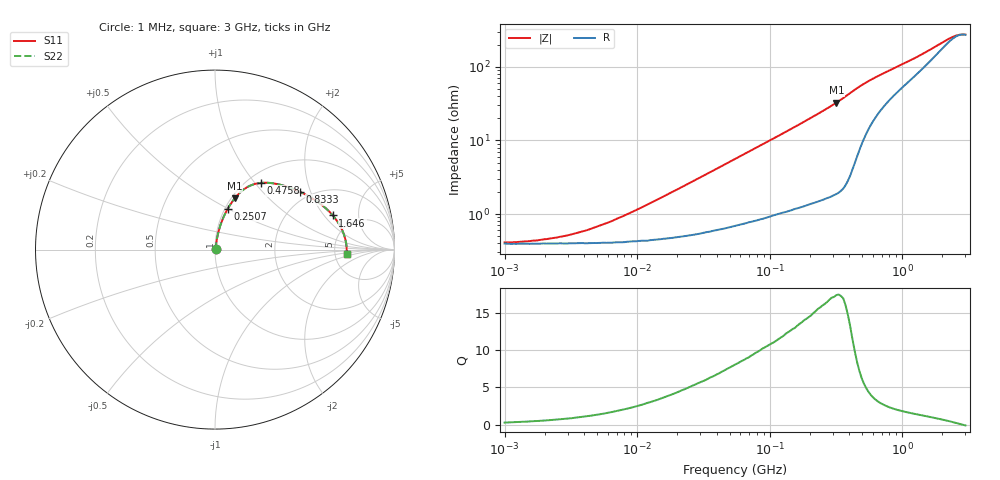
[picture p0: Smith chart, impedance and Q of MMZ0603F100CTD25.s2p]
! S-Parameter Data Generated by TDK Corporation
! Copyright(C) 2025 TDK Corporation.
! All Rights Reserved.
! TDK P/N: MMZ0603F100CTD25 (Chip Bead)
! Property: |Z|=10ohm at 100MHz
! Size(LxWxT): 0.6x0.3x0.3mm
! Model Type: s2p (Touchstone File Format Version 1.0)
! Frequency: DC=Yes Start=1MHz Stop=3000MHz 202points Log-sweep
! Model Generated on Feb. 6, 2025
! Terms and conditions regarding TDK Simulation Models:
! 1)This simulation model is being provided solely for informational
!  purposes. Please refer to the specifications of the products in
!  terms of detailed characteristics of such products.
! 2)In no event shall TDK Corporation of any of its subsidiaries be
!  liable for any loss or damage arising, directly or indirectly,
!  from any information contained in this simulation model, including,
!  but not limited to loss or damages arising from any inaccuracies,
!  omissions or errors in connection with such information.
! 3)Any and all copyrights on this simulation model are owned by
!  TDK Corporation.  Duplication or redistribution of this simulation
!  model without prior written permission from TDK Corporation
!  is prohibited.
! 4)This simulation model is subject to any modification or change
!  without any prior notice.
! 5)Neither TDK Corporation nor any of its subsidiaries shall make any
!  warranty, express or implied, including but not limited to the
!  correctness, implied warranties of merchantability and fitness for
!  a particular purpose with respect to this simulation models.
! 6)The use of this simulation model shall be deemed to have consented
!  to the terms and conditions hereof.
! Port Assignments:
!  1 ---@@@--- 2
! Applicable Conditions:
!  Temperature = 25 degC
!  DC Bias Current = 0 A
!  Small Signal Operation
# Hz S MA R 50
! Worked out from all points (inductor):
!   201 points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, 1 MHz to 3 GHz, reference 50 ohm
!   read as one part in series: L = 16.8 nH near 12.45 MHz
!   highest Q = 17.3 at 318.8 MHz (marker M1), where L = 16.3 nH
!   self-resonance near 2.843 GHz
!   S11 on the Smith chart (normalised r, x): 1 MHz: 1.01, +0.00; 250.7 MHz: 1.03, +0.50; 475.8 MHz: 1.15, +1.07; 833.3 MHz: 1.76, +1.69; 1.646 GHz: 3.45, +2.47; 3 GHz: 6.46, -0.63
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1000000  0.004095 15.2  0.996 -0.1  0.996 -0.1  0.004095 15.2
1221597  0.004115 18.1  0.9961 -0.1  0.9961 -0.1  0.004115 18.1
2139570  0.004579 30.1  0.996 -0.1  0.996 -0.1  0.004579 30.1
2947212  0.005076 38.6  0.996 -0.2  0.996 -0.2  0.005076 38.6
3900413  0.0058 46.0  0.996 -0.2  0.996 -0.2  0.0058 46.0
6305767  0.007855 58.5  0.9959 -0.4  0.9959 -0.4  0.007855 58.5
1.461624e7  0.01607 72.8  0.9954 -0.9  0.9954 -0.9  0.01607 72.8
5.477226e7  0.05539 79.8  0.9917 -3.2  0.9917 -3.2  0.05539 79.8
1.171891e8  0.1144 78.5  0.9836 -6.5  0.9836 -6.5  0.1144 78.5
2.136344e8  0.2042 74.4  0.9655 -11.8  0.9655 -11.8  0.2042 74.4
2.507343e8  0.2391 72.6  0.9562 -13.8  0.9562 -13.8  0.2391 72.6
3.188066e8  0.305 69.0  0.935 -17.7  0.935 -17.7  0.305 69.0
3.894533e8  0.3771 64.0  0.901 -22.1  0.901 -22.1  0.3771 64.0
4.75755e8  0.4499 55.6  0.8334 -26.5  0.8334 -26.5  0.4499 55.6
6.049187e8  0.5109 45.1  0.735 -29.5  0.735 -29.5  0.5109 45.1
8.005644e8  0.5649 35.5  0.6319 -31.3  0.6319 -31.3  0.5649 35.5
8.332625e8  0.5719 34.3  0.6182 -31.4  0.6182 -31.4  0.5719 34.3
1.243477e9  0.6395 23.6  0.4864 -31.7  0.4864 -31.7  0.6395 23.6
1.645649e9  0.6834 16.2  0.393 -29.0  0.393 -29.0  0.6834 16.2
2.455801e9  0.7282 4.6  0.2804 -12.1  0.2804 -12.1  0.7282 4.6
2.660507e9  0.7324 2.1  0.2695 -5.8  0.2695 -5.8  0.7324 2.1
3e9  0.7341 -1.8  0.2672 4.8  0.2672 4.8  0.7341 -1.8
